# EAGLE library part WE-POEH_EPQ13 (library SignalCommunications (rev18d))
WE-PoEH Power over Ethernet High Power Transformer Characteristics DFlyback or Forward Transformer Input voltage: 9 V or 33 V to 57 V Switching frequencies: 200-400 kHz Operating temperature: -40°C up to +125°C Insulation test voltage: 1.5 kVAC Different output voltages available Optimized core and bobbin design for 30% more power handling Standard footprint to EP13 Applications PoE and PoE+ powered devices Telecom Industrial applications WLAN acess point Safety cameras Details see: http://katalog.we-online.de/en/pbs/WE-POEH 20146 (C) Wurth Elektronik
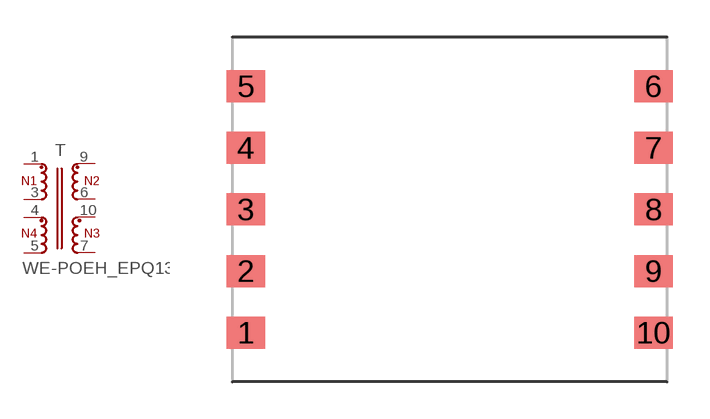
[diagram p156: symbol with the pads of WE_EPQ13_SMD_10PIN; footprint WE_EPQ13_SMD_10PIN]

Designator prefix T

## WE-POEH_EPQ13_7491195112, WE-POEH_EPQ13_7491195212, WE-POEH_EPQ13_7491195224, WE-POEH_EPQ13_749119533, WE-POEH_EPQ13_7491195331, WE-POEH_EPQ13_749119550, WE-POEH_EPQ13_7491195501, WE-POEH_EPQ13_7491196112, WE-POEH_EPQ13_7491196212, WE-POEH_EPQ13_749119633, WE-POEH_EPQ13_7491196331, WE-POEH_EPQ13_749119650, WE-POEH_EPQ13_7491196501  [WE_EPQ13_SMD_10PIN]
1  1  pas
3  8  pas
4  7  pas
5  6  pas
6  3  pas
7  5  pas
9  2  pas
10  4  pas

## Footprint WE_EPQ13_SMD_10PIN (pad centres in mm)
smd 1.55 x 1.3: 1 -8.275,-5; 2 -8.275,-2.5; 3 -8.275,0; 4 -8.275,2.5; 5 -8.275,5; 6 8.275,5; 7 8.275,2.5; 8 8.275,0; 9 8.275,-2.5; 10 8.275,-5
